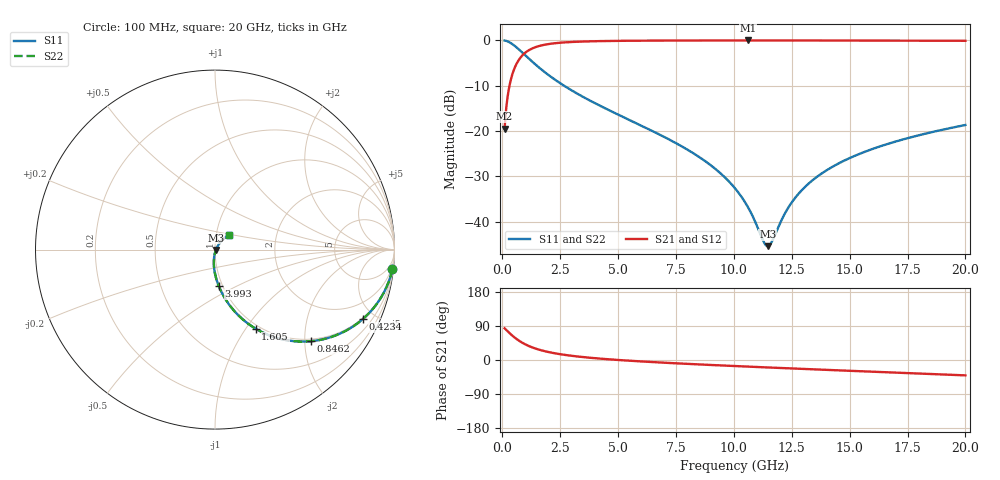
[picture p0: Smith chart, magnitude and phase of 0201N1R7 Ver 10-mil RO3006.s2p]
# GHz S MA R 50
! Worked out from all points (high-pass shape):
!   1601 points, 100 MHz to 20 GHz, reference 50 ohm
!   highest |S21| = -0.05 dB at 10.61 GHz (marker M1); lowest = -19.5 dB at 100 MHz (marker M2)
!   |S21| within 3 dB of the highest: 924.7 MHz to end of sweep
!   lowest |S11| = -45.4 dB at 11.47 GHz (marker M3), VSWR 1.01, Z = 50.5 - j0.182 ohm
!   |S11| at or under -10 dB: 2.659 GHz to end of sweep
!   |S22| runs from -45.4 to 0.0 dB; largest |S21 - S12| = 0
!   S11 on the Smith chart (normalised r, x): 100 MHz: 1, -18; 423.4 MHz: 0.95, -4.29; 846.2 MHz: 0.95, -2.14; 1.605 GHz: 0.95, -1.11; 3.993 GHz: 0.96, -0.40; 20 GHz: 1.16, +0.20
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0.1  0.9943 -6.3  0.1062 83.7  0.1062 83.7  0.9943 -6.3
0.274125  0.9595 -16.8  0.2812 73.2  0.2812 73.2  0.9595 -16.8
0.423375  0.9105 -25.1  0.4124 64.8  0.4124 64.8  0.9105 -25.1
0.6099375  0.8365 -34.2  0.5466 55.7  0.5466 55.7  0.8365 -34.2
0.84625  0.7392 -43.7  0.6717 46.2  0.6717 46.2  0.7392 -43.7
1.206937  0.6078 -54.5  0.7919 35.3  0.7919 35.3  0.6078 -54.5
1.604937  0.4958 -62.8  0.8659 26.9  0.8659 26.9  0.4958 -62.8
2.33875  0.3581 -72.6  0.9306 16.9  0.9306 16.9  0.3581 -72.6
3.420812  0.2427 -81.1  0.9666 8.1  0.9666 8.1  0.2427 -81.1
3.992938  0.2029 -84.2  0.9755 4.8  0.9755 4.8  0.2029 -84.2
6.741625  0.09262 -93.6  0.9911 -6.3  0.9911 -6.3  0.09262 -93.6
8.744063  0.04682 -96.5  0.9939 -12.4  0.9939 -12.4  0.04682 -96.5
10.05  0.02334 -93.4  0.9944 -16.0  0.9944 -16.0  0.02334 -93.4
10.60969  0.01445 -86.4  0.9944 -17.5  0.9944 -17.5  0.01445 -86.4
11.28131  0.00605 -47.4  0.9944 -19.2  0.9944 -19.2  0.00605 -47.4
11.46787  0.005367 -19.6  0.9943 -19.7  0.9943 -19.7  0.005367 -19.6
11.642  0.006014 6.0  0.9943 -20.1  0.9943 -20.1  0.006014 6.0
12.46288  0.01577 47.2  0.994 -22.2  0.994 -22.2  0.01577 47.2
13.37081  0.02823 53.8  0.9936 -24.5  0.9936 -24.5  0.02823 53.8
14.76381  0.04706 54.8  0.9926 -27.9  0.9926 -27.9  0.04706 54.8
16.69162  0.07255 52.4  0.9907 -32.6  0.9907 -32.6  0.07255 52.4
20  0.1163 46.0  0.9858 -40.6  0.9858 -40.6  0.1163 46.0
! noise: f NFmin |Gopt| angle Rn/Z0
0.1  0.0009681  0.9571  0.7136  0.005079
2.301  0.005359  0.826  4.396  0.006466
4.515  0.008286  0.7844  8.109  0.007856
6.729  0.01081  0.7578  11.82  0.008936
8.943  0.01311  0.7383  15.52  0.009852
11.14  0.01527  0.7234  19.16  0.01066
13.36  0.01735  0.7114  22.79  0.0114
15.57  0.01937  0.7018  26.38  0.01208
17.79  0.02134  0.694  29.92  0.01273
20  0.0233  0.6877  33.42  0.01334
